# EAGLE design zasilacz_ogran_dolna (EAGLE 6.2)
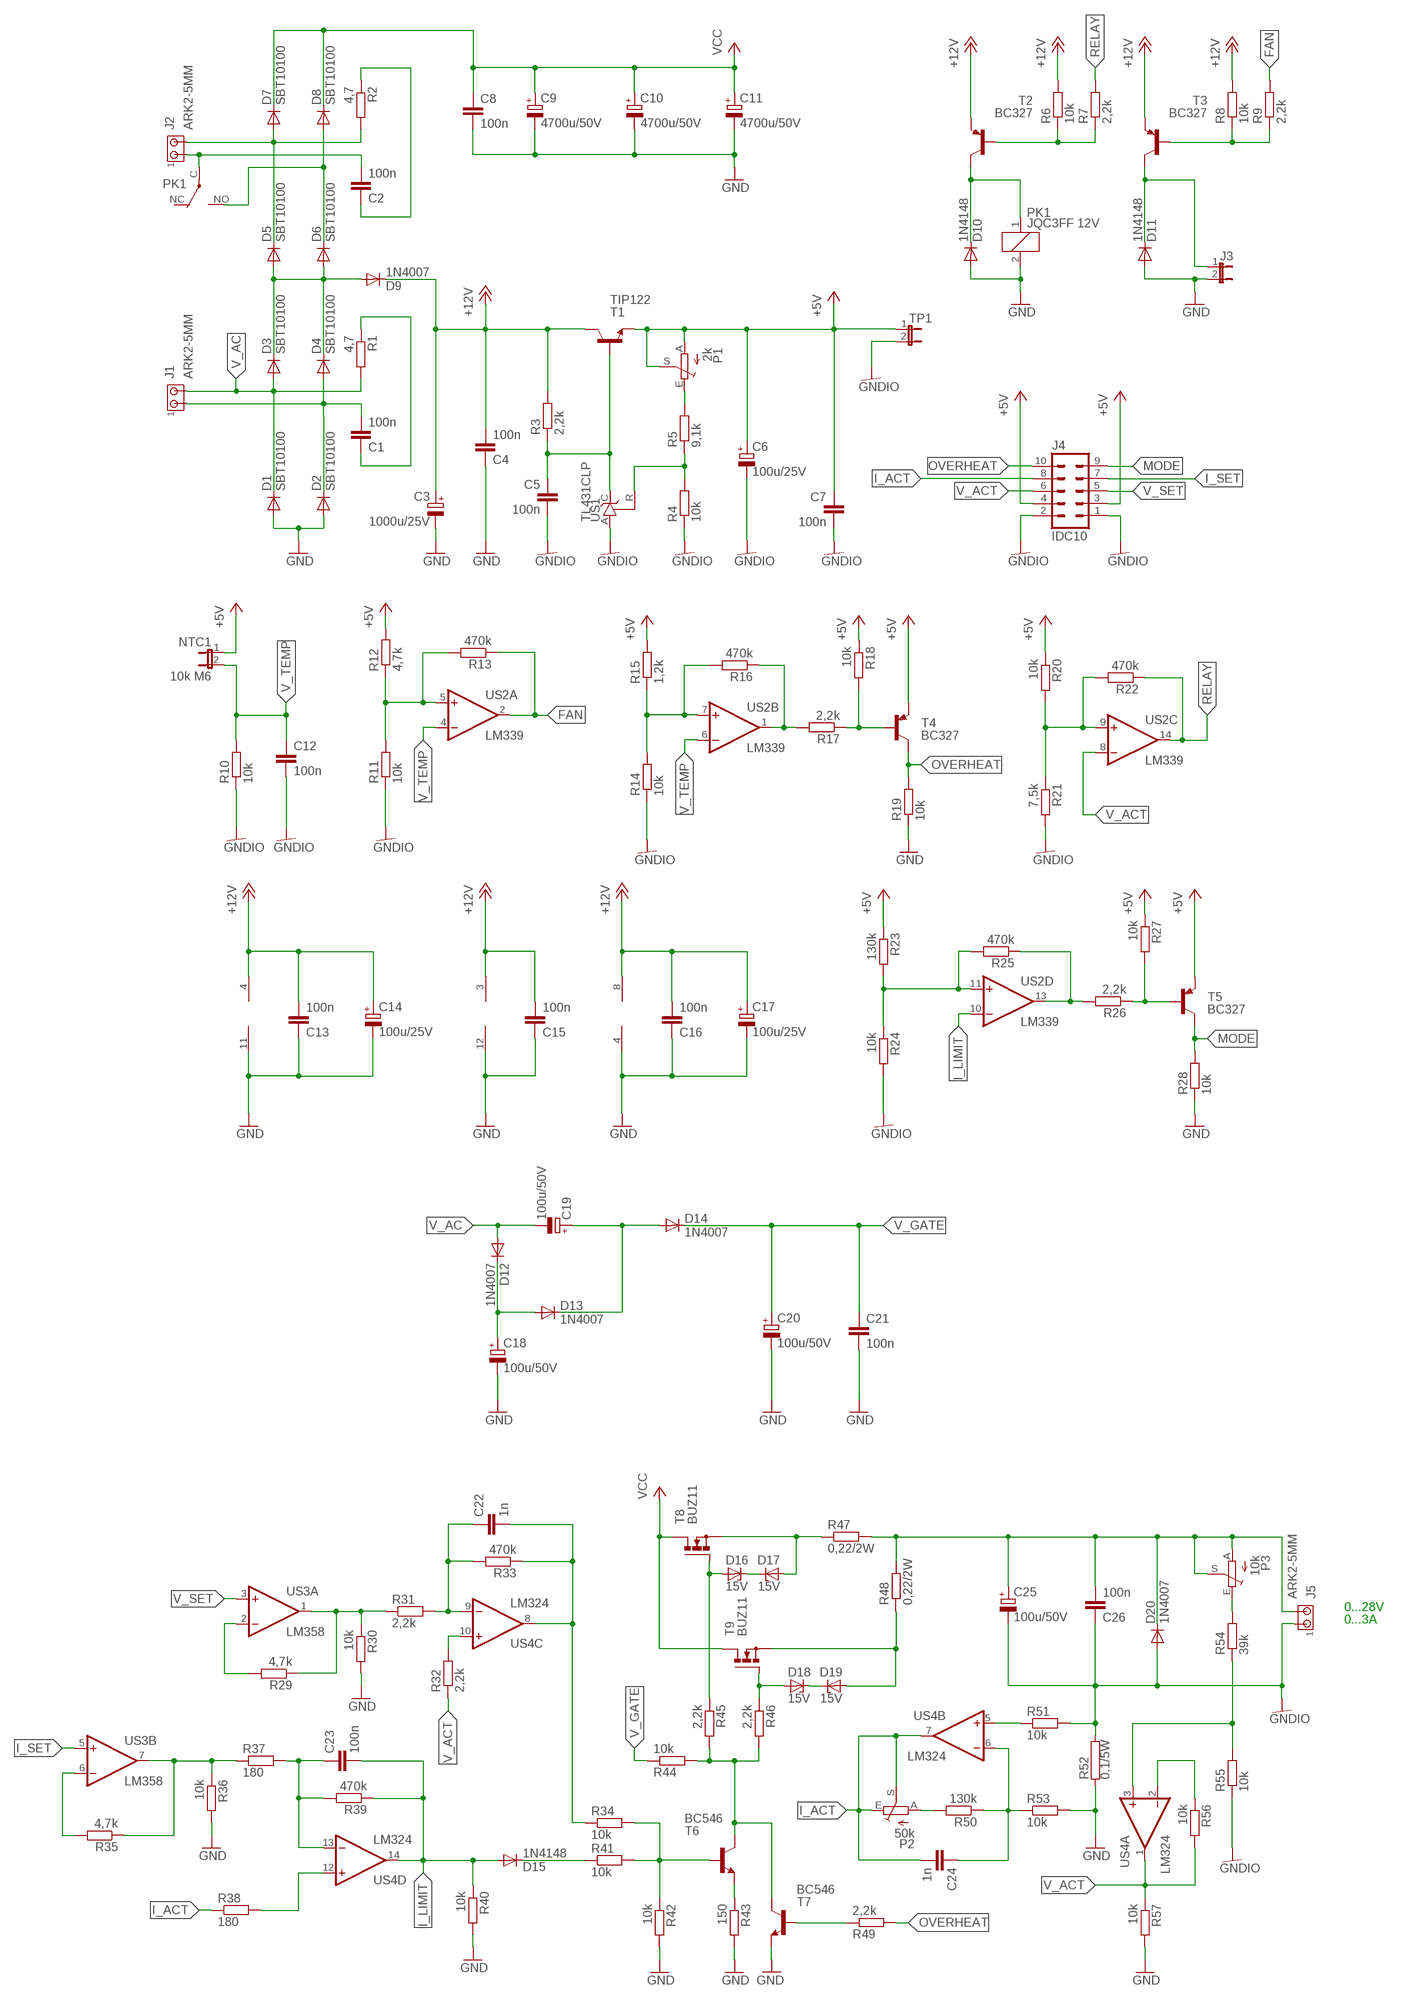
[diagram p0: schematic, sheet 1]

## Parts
C1  100n  C-EU050-025X075  [C050-025X075]
C2  100n  C-EU050-025X075  [C050-025X075]
C3  1000u/25V  CPOL-EUE5-10.5  [E5-10,5]
C4  100n  C-EU050-025X075  [C050-025X075]
C5  100n  C-EU050-025X075  [C050-025X075]
C6  100u/25V  CPOL-EUE2.5-6  [E2,5-6]
C7  100n  C-EU050-025X075  [C050-025X075]
C8  100n  C-EU050-025X075  [C050-025X075]
C9  4700u/50V  CPOL-EUE10-20  [EB20D]
C10  4700u/50V  CPOL-EUE10-20  [EB20D]
C11  4700u/50V  CPOL-EUE10-20  [EB20D]
C12  100n  C-EU050-025X075  [C050-025X075]
C13  100n  C-EU050-025X075  [C050-025X075]
C14  100u/25V  CPOL-EUE2.5-6  [E2,5-6]
C15  100n  C-EU050-025X075  [C050-025X075]
C16  100n  C-EU050-025X075  [C050-025X075]
C17  100u/25V  CPOL-EUE2.5-6  [E2,5-6]
C18  100u/50V  CPOL-EUE3.5-8  [E3,5-8]
C19  100u/50V  CPOL-EUE3.5-8  [E3,5-8]
C20  100u/50V  CPOL-EUE3.5-8  [E3,5-8]
C21  100n  C-EU050-025X075  [C050-025X075]
C22  1n  C-EU050-025X075  [C050-025X075]
C23  100n  C-EU050-025X075  [C050-025X075]
C24  1n  C-EU050-025X075  [C050-025X075]
C25  100u/50V  CPOL-EUE3.5-8  [E3,5-8]
C26  100n  C-EU050-025X075  [C050-025X075]
D1  SBT10100  DIODE-TO220V  [TO220ACS]
D2  SBT10100  DIODE-TO220V  [TO220ACS]
D3  SBT10100  DIODE-TO220V  [TO220ACS]
D4  SBT10100  DIODE-TO220V  [TO220ACS]
D5  SBT10100  DIODE-TO220V  [TO220ACS]
D6  SBT10100  DIODE-TO220V  [TO220ACS]
D7  SBT10100  DIODE-TO220V  [TO220ACS]
D8  SBT10100  DIODE-TO220V  [TO220ACS]
D9  1N4007  DIODE-DO41-7.6  [DO41-7.6]
D10  1N4148  DIODE-DO34-7  [DO34-7]
D11  1N4148  DIODE-D-5  [D-5]
D12  1N4007  1N4004  [DO41-10]
D13  1N4007  1N4004  [DO41-10]
D14  1N4007  1N4004  [DO41-10]
D15  1N4148  DIODE-DO34-7  [DO34-7]
D16  15V  ZENER-DIODEDO34-7  [DO34Z7]
D17  15V  ZENER-DIODEDO34-7  [DO34Z7]
D18  15V  ZENER-DIODEDO34-7  [DO34Z7]
D19  15V  ZENER-DIODEDO34-7  [DO34Z7]
D20  1N4007  DIODE-DO41-7.6  [DO41-7.6]
J1  ARK2-5MM  [2PIN-5MM]
J2  ARK2-5MM  [2PIN-5MM]
J3  JP1E  [JP1]
J4  IDC10  ML10  [ML10]
J5  ARK2-5MM  [2PIN-5MM]
NTC1  10k M6  JP1E  [JP1]
P1  2k  TRIM_EU-B64Y  [B64Y]
P2  50k  TRIM_EU-B64Y  [B64Y]
P3  10k  TRIM_EU-B64Y  [B64Y]
PK1  JQC3FF 12V  PK_POJED-JQC-3FG  [PK_POJED_JQC-3FG]
R1  4,7  R-EU_0207/7  [0207/7]
R2  4,7  R-EU_0207/7  [0207/7]
R3  2,2k  R-EU_0207/7  [0207/7]
R4  10k  R-EU_0207/7  [0207/7]
R5  9,1k  R-EU_0207/7  [0207/7]
R6  10k  R-EU_0207/7  [0207/7]
R7  2,2k  R-EU_0207/7  [0207/7]
R8  10k  R-EU_0207/7  [0207/7]
R9  2,2k  R-EU_0207/7  [0207/7]
R10  10k  R-EU_0207/7  [0207/7]
R11  10k  R-EU_0207/7  [0207/7]
R12  4,7k  R-EU_0207/7  [0207/7]
R13  470k  R-EU_0207/7  [0207/7]
R14  10k  R-EU_0207/7  [0207/7]
R15  1,2k  R-EU_0207/7  [0207/7]
R16  470k  R-EU_0207/7  [0207/7]
R17  2,2k  R-EU_0207/7  [0207/7]
R18  10k  R-EU_0207/7  [0207/7]
R19  10k  R-EU_0207/7  [0207/7]
R20  10k  R-EU_0207/7  [0207/7]
R21  7,5k  R-EU_0207/7  [0207/7]
R22  470k  R-EU_0207/7  [0207/7]
R23  130k  R-EU_0207/7  [0207/7]
R24  10k  R-EU_0207/7  [0207/7]
R25  470k  R-EU_0207/7  [0207/7]
R26  2,2k  R-EU_0207/7  [0207/7]
R27  10k  R-EU_0207/7  [0207/7]
R28  10k  R-EU_0207/7  [0207/7]
R29  4,7k  R-EU_0207/7  [0207/7]
R30  10k  R-EU_0207/7  [0207/7]
R31  2,2k  R-EU_0207/7  [0207/7]
R32  2,2k  R-EU_0207/7  [0207/7]
R33  470k  R-EU_0207/7  [0207/7]
R34  10k  R-EU_0207/7  [0207/7]
R35  4,7k  R-EU_0207/7  [0207/7]
R36  10k  R-EU_0207/7  [0207/7]
R37  180  R-EU_0207/7  [0207/7]
R38  180  R-EU_0207/7  [0207/7]
R39  470k  R-EU_0207/7  [0207/7]
R40  10k  R-EU_0207/7  [0207/7]
R41  10k  R-EU_0207/7  [0207/7]
R42  10k  R-EU_0207/7  [0207/7]
R43  150  R-EU_0207/7  [0207/7]
R44  10k  R-EU_0207/7  [0207/7]
R45  2,2k  R-EU_0207/7  [0207/7]
R46  2,2k  R-EU_0207/7  [0207/7]
R47  0,22/2W  R-EU_0817/7V  [P0817V]
R48  0,22/2W  R-EU_0817/7V  [P0817V]
R49  2,2k  R-EU_0207/7  [0207/7]
R50  130k  R-EU_0207/7  [0207/7]
R51  10k  R-EU_0207/7  [0207/7]
R52  0,1/5W  R-5W  [R_5W]
R53  10k  R-EU_0207/7  [0207/7]
R54  39k  R-EU_0207/7  [0207/7]
R55  10k  R-EU_0207/7  [0207/7]
R56  10k  R-EU_0207/7  [0207/7]
R57  10k  R-EU_0207/7  [0207/7]
T1  TIP122  -NPN-TO220V  [TO220V]
T2  BC327  BC556  [TO92-EBC]
T3  BC327  BC556  [TO92-EBC]
T4  BC327  BC556  [TO92-EBC]
T5  BC327  BC556  [TO92-EBC]
T6  BC546  BC546A  [TO92-EBC]
T7  BC546  BC546A  [TO92-EBC]
T8  BUZ11  BUZ11BV  [TO220BV]
T9  BUZ11  BUZ11BV  [TO220BV]
TP1  JP1E  [JP1]
US1  TL431CLP  [TO92-CLP]
US2  LM339  LM339N  [DIL14]
US3  LM358  LM358N  [DIL08]
US4  LM324  LM324N  [DIL14]

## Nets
+5V: C6.+ C7.1 J4.3 J4.4 NTC1.1 P1.A P1.S R12.2 R15.2 R18.1 R20.1 R23.1 R27.1 T1.3(E) T4.E T5.E TP1.1
+12V: C3.+ C4.2 C13.2 C14.+ C15.2 C16.2 C17.+ D9.C R3.2 R6.2 R8.2 T1.2(C) T2.E T3.E US2.3(P:V+) US3.8(P:V+) US4.4(P:V+)
FAN: R9.2 R13.1 US2.2(A:OUT)
GND: C3.- C4.1 C8.2 C9.- C10.- C11.- C13.1 C14.- C15.1 C16.1 C17.- C18.- C20.- C21.2 D1.A D2.A D10.A D11.A J3.2 PK1.2 R19.1 R28.1 R30.2 R36.2 R40.2 R42.2 R43.2 R52.P$1 R53.2 R57.2 T7.E US2.12(P:GND) US3.4(P:V-) US4.11(P:V-)
GNDIO: C5.2 C6.- C7.2 C12.2 C25.- C26.1 D20.A J4.1 J4.2 J5.P$1 R4.1 R10.1 R11.1 R14.1 R21.2 R24.2 R51.2 R52.P$2 R55.1 TP1.2 US1.A
I_ACT: C24.2 J4.8 P2.E P2.S R38.1 US4.7(B:OUT)
I_LIMIT: C23.2 D15.A R39.1 R40.1 US2.10(D:-IN) US4.14(D:OUT)
I_SET: J4.7 US3.5(B:+IN)
MODE: J4.9 R28.2 T5.C
N$1: D17.A R47.1 T8.S
N$2: R16.1 R17.2 US2.1(B:OUT)
N$3: C1.1 R1.1
N$4: R11.2 R12.1 R13.2 US2.5(A:+IN)
N$5: R17.1 R18.2 T4.B
N$6: R14.2 R15.1 R16.2 US2.7(B:+IN)
N$7: D19.A R48.1 T9.S
N$8: C5.1 R3.1 T1.1(B) US1.C
N$9: C19.+ D13.C D14.A
N$10: C1.2 D2.C D4.A J1.P$1
N$11: C25.+ C26.2 D20.C J5.P$2 P3.A P3.S R47.2 R48.2
N$12: C18.+ D12.C D13.A
N$13: D16.A R45.1 T8.G
N$14: P3.E R54.2
N$15: D15.C R41.1
N$16: C22.1 R31.2 R33.2 US4.9(C:-IN)
N$17: C24.1 R50.1 R53.1 US4.6(B:-IN)
N$18: P2.A R50.2
N$19: R43.1 T6.E
N$20: C22.2 R33.1 R34.1 US4.8(C:OUT)
N$21: R54.1 R55.2 US4.3(A:+IN)
N$22: R32.2 US4.10(C:+IN)
N$23: P1.E R5.2
N$24: C2.1 R2.1
N$25: D10.C PK1.1 T2.C
N$26: D3.C D4.C D5.A D6.A D9.A
N$27: D5.C D7.A J2.P$2 R2.2
N$28: D6.C D8.A PK1.NO
N$29: R6.1 R7.1 T2.B
N$30: D11.C J3.1 T3.C
N$31: C2.2 J2.P$1 PK1.C(COM)
N$32: R8.1 R9.1 T3.B
N$33: R4.2 R5.1 US1.R
N$35: R49.1 T7.B
N$36: C23.1 R37.2 R39.2 US4.13(D:-IN)
N$37: R25.1 R26.2 US2.13(D:OUT)
N$39: R26.1 R27.2 T5.B
N$40: R23.2 R24.1 R25.2 US2.11(D:+IN)
N$41: R20.2 R21.1 R22.2 US2.9(C:+IN)
N$47: D16.C D17.C
N$48: R44.2 R45.2 R46.2 T6.C T7.C
N$49: D18.A R46.1 T9.G
N$50: D18.C D19.C
N$52: R34.2 R41.2 R42.1 T6.B
N$53: R51.1 US4.5(B:+IN)
N$54: R29.2 US3.2(A:-IN)
N$58: R38.2 US4.12(D:+IN)
N$59: R35.2 US3.6(B:-IN)
N$60: R29.1 R30.1 R31.1 US3.1(A:OUT)
N$61: R56.1 US4.2(A:-IN)
N$62: R35.1 R36.1 R37.1 US3.7(B:OUT)
OVERHEAT: J4.10 R19.2 R49.2 T4.C
RELAY: R7.2 R22.1 US2.14(C:OUT)
V_AC: C19.- D1.C D3.A D12.A J1.P$2 R1.2
V_ACT: J4.6 R32.1 R56.2 R57.1 US2.8(C:-IN) US4.1(A:OUT)
V_GATE: C20.+ C21.1 D14.C R44.1
V_SET: J4.5 US3.3(A:+IN)
V_TEMP: C12.1 NTC1.2 R10.2 US2.4(A:-IN) US2.6(B:-IN)
VCC: C8.1 C9.+ C10.+ C11.+ D7.C D8.C T8.D T9.D
Unconnected: PK1.NC

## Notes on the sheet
- 0...28V
- 0...3A

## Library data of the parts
C1 C2 C4 C5 C7 C8 C12 C13 C15 C16 C21-C24 C26 = rcl:C-EU: CAPACITOR, European symbol
C3 C6 C9-C11 C14 C17-C20 C25 = rcl:CPOL-EU: POLARIZED CAPACITOR, European symbol
D1-D11 D15 D20 = diode:DIODE-: DIODE
D12-D14 = diode:1N4004: DIODE
D16-D19 = diode:ZENER-DIODE: Z-Diode
J1 J2 J5 = zlacza_futrzak:ARK2: ARK 2
J3 NTC1 TP1 = jumper:JP1E: JUMPER
J4 = con-ml:ML10: HARTING; OC_FARNELL: unknown; OC_NEWARK: unknown
P1-P3 = pot:TRIM_EU-: POTENTIOMETER
PK1 = inne_futrzak:PK_POJED
R1-R51 R53-R57 = rcl:R-EU_: RESISTOR, European symbol
R52 = inne_futrzak:R
T1 = transistor:*-NPN-: NPN Transistror BF959 corrected 2008.03.06
T2-T5 = transistor-pnp:BC556*: PNP Transistror
T6 T7 = transistor-npn:BC546*: NPN Transistor
T8 T9 = transistor-power:BUZ11: N-CHANNEL MOS FET
US1 = v-reg:TL431CLP: VOLTAGE REGULATOR
US2 = linear:LM339: Low Power Low Offset Voltage Quad Comparators with open collector; LM139/LM239/LM339/LM2901/LM3302
US3 = linear:LM358: OP AMP also LM158; LM258; LM2904 Source: http://cache.national.com/ds/LM/LM158.pdf
US4 = linear:LM324: OP AMP

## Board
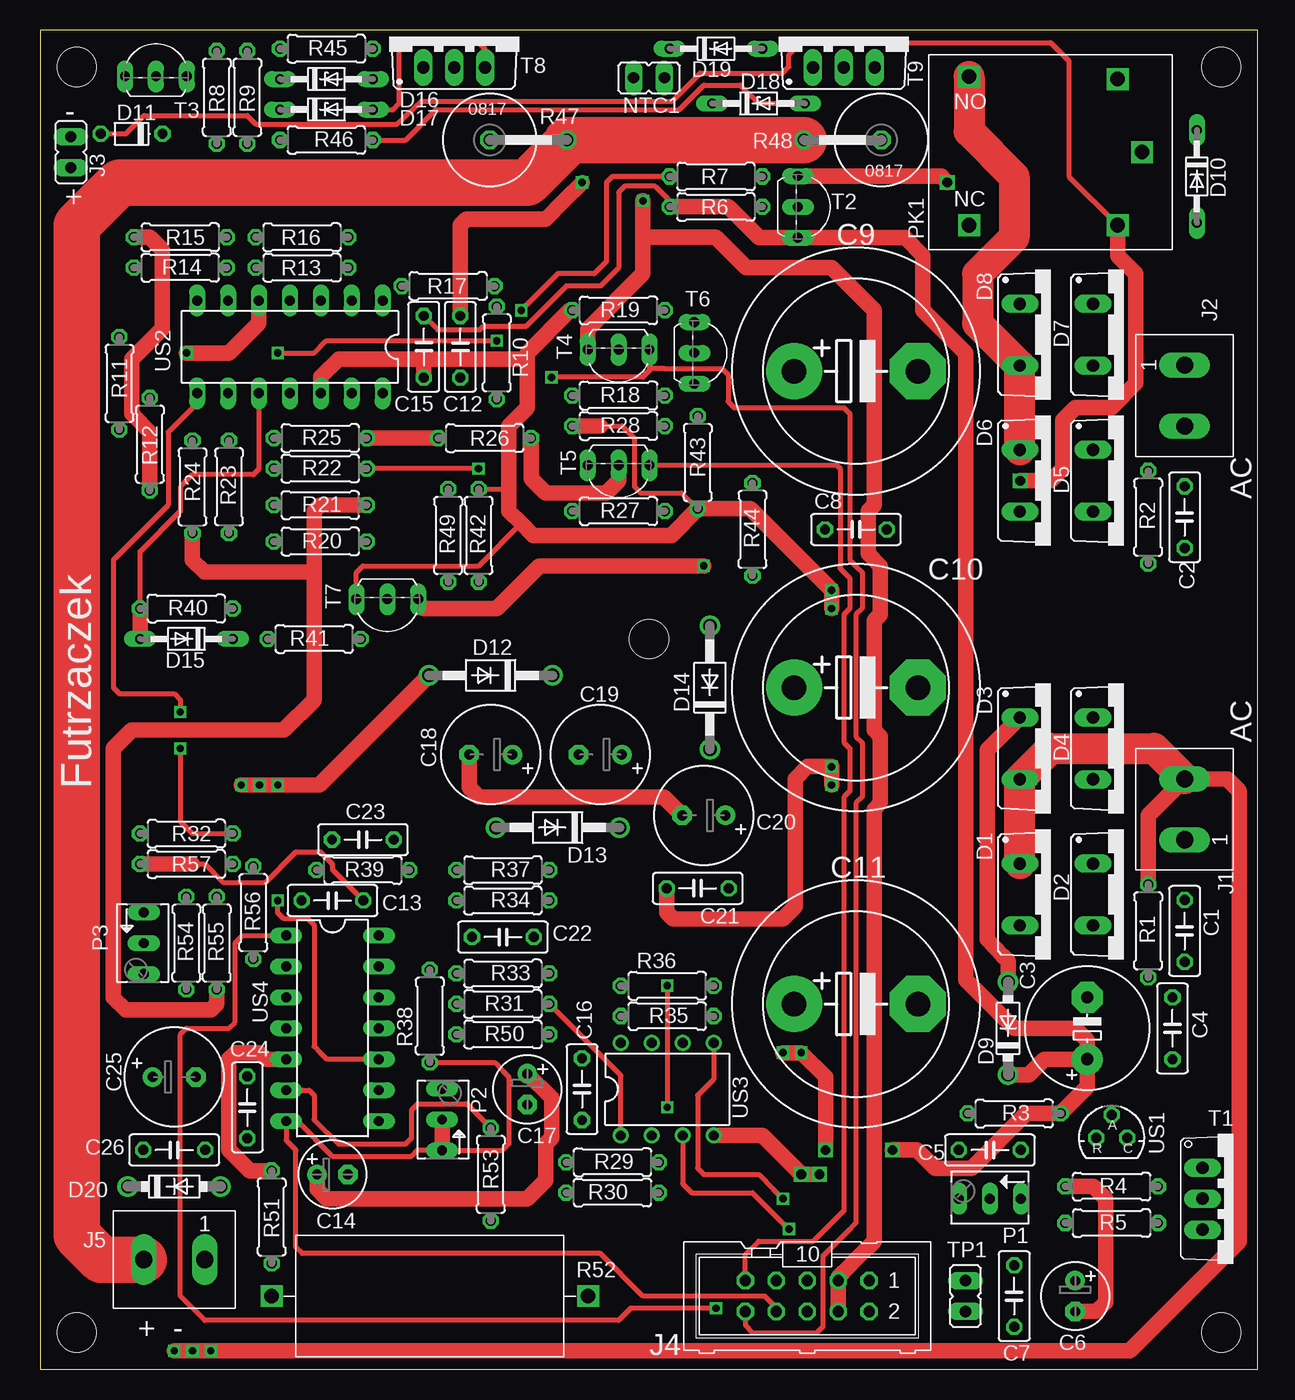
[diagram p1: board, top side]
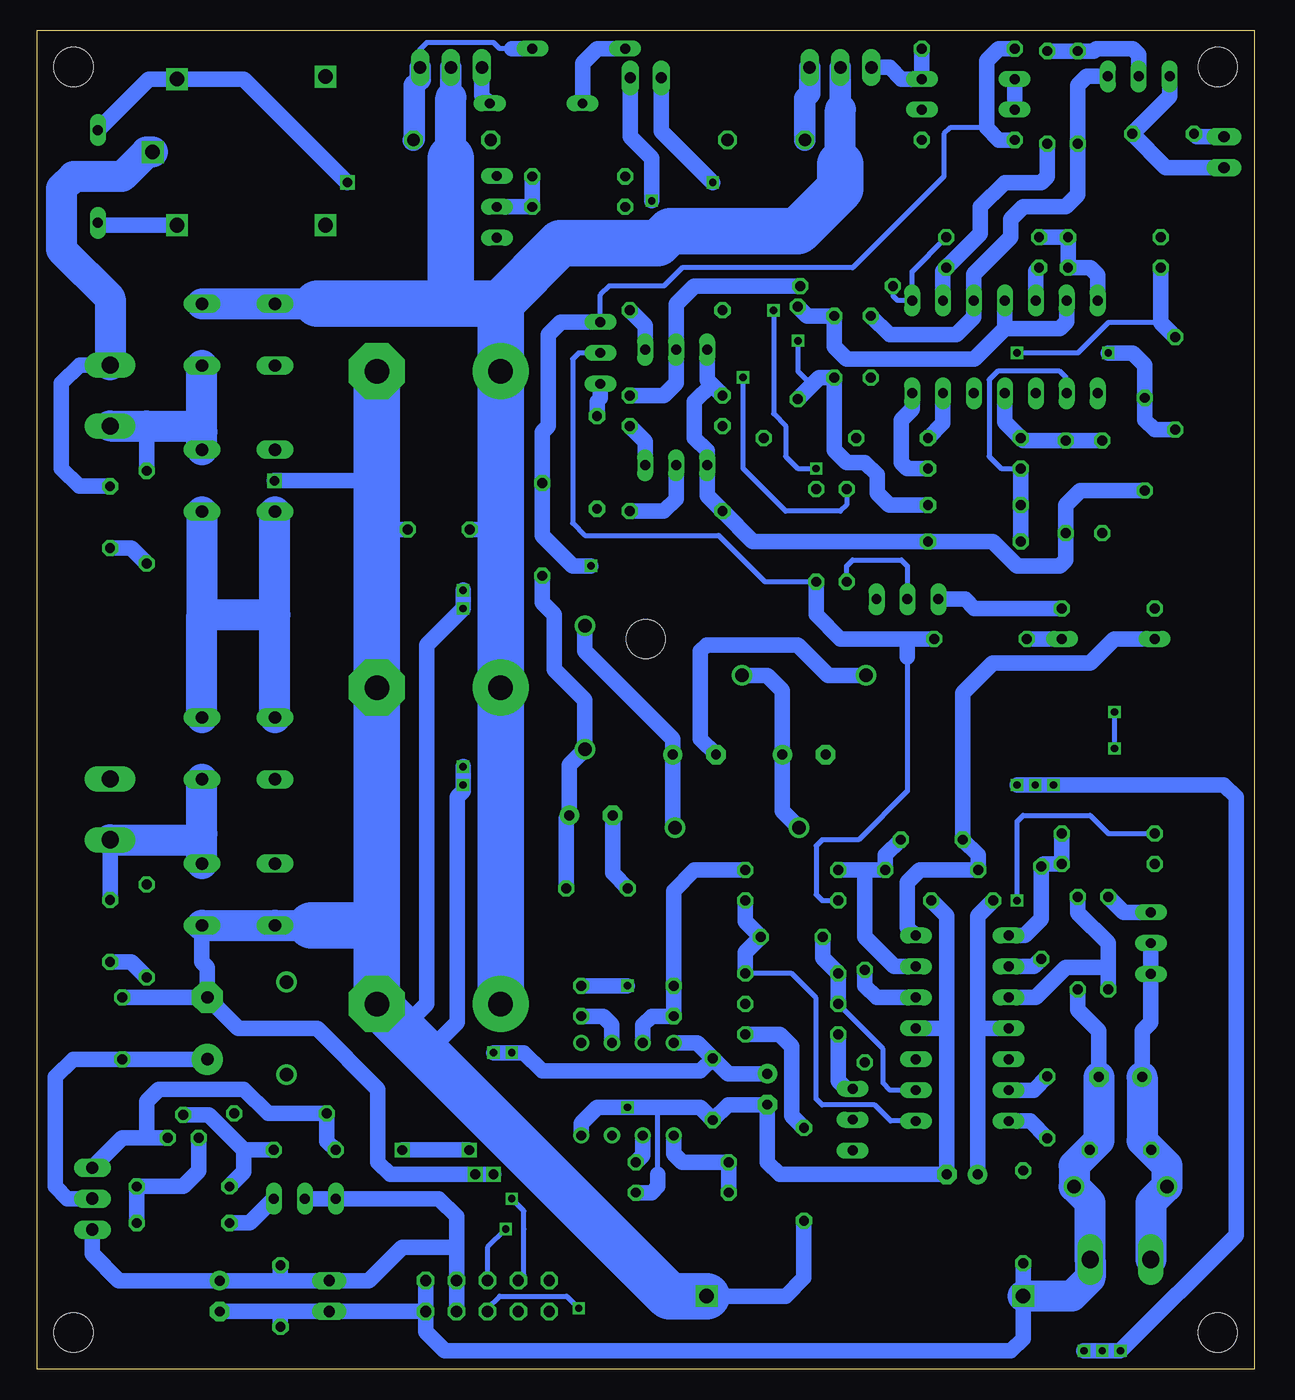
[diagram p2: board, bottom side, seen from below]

Size 100 x 110 mm. Coordinates in mm from the lower left corner, seen from the top.
Outline: 0,0 100,0 100,110 0,110 0,0
Copper layers (1*16): Top 0.035mm / dielectric 1.5mm / Bottom 0.035mm
Design rules: minimum track width 10mil, minimum drill 23mil, track to track 8mil, track to pad 8mil, pad to pad 8mil, via to via 8mil, smd to smd 8mil, copper to edge 20mil, drill to drill 8mil, minimum pad ring 10mil, minimum via ring 8mil, stop-mask expansion 4mil, vias tented up to drill 0mil, thermal gap 10mil
Holes 3.2 mm at 3,3 97,3 3,107 97,107 50,60

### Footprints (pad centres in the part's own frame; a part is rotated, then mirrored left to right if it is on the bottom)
C050-025X075 = drill 0.813 octagon: 1 -2.54,0; 2 2.54,0
E5-10,5 = drill 1.016 pad 2.54: + -2.54,0 | drill 1.016 pad 2.54 octagon: - 2.54,0
E2,5-6 = drill 0.813 pad 1.6: + -1.27,0 | drill 0.813 pad 1.6 octagon: - 1.27,0
EB20D = drill 2.007 pad 4.597: + -5.08,0 | drill 2.007 pad 4.597 octagon: - 5.08,0
E3,5-8 = drill 0.813 pad 1.6: + -1.778,0 | drill 0.813 pad 1.6 octagon: - 1.778,0
TO220ACS = drill 1.016 long: A 2.54,-2.54; C -2.54,-2.54
DO41-7.6 = drill 1.1 pad 1.7: A 3.81,0; C -3.81,0
DO34-7 = drill 0.813 long: A 3.81,0; C -3.81,0
D-5 = drill 0.813 octagon: A 2.54,0; C -2.54,0
DO41-10 = drill 1.118: A 5.08,0; C -5.08,0
DO34Z7 = drill 0.813 long: A 3.81,0; C -3.81,0
2PIN-5MM = drill 1.4 long: P$1 -2.5,0; P$2 2.5,0
JP1 = drill 0.914 long: 1 0,-1.27; 2 0,1.27
ML10 = drill 0.914 octagon: 1 -5.08,-1.27; 2 -5.08,1.27; 3 -2.54,-1.27; 4 -2.54,1.27; 5 0,-1.27; 6 0,1.27; 7 2.54,-1.27; 8 2.54,1.27; 9 5.08,-1.27; 10 5.08,1.27
B64Y = drill 0.813 long: A 2.54,0; E -2.54,0; S 0,0
PK_POJED_JQC-3FG = drill 1.2 square: 1 5.5,6; 2 5.5,-6; C 7.5,0; NC -6.7,-6; NO -6.7,6.2
0207/7 = drill 0.813 octagon: 1 -3.81,0; 2 3.81,0
P0817V = drill 1.016 octagon: 1 -5.08,0; 2 1.27,0
R_5W = drill 1.2 square: P$1 -13,0; P$2 13,0
TO220V = drill 1.016 long: 1 -2.54,-2.54; 2 0,-2.54; 3 2.54,-2.54
TO92-EBC = drill 0.813 long: B 0,-1.27; C -2.54,-1.27; E 2.54,-1.27
TO220BV = drill 1.016 long: D 0,-2.54; G -2.54,-2.54; S 2.54,-2.54
TO92-CLP = drill 0.813 octagon: A 0,1.905; C 1.27,0; R -1.27,0
DIL14 = drill 0.813 long: 1 -7.62,-3.81; 2 -5.08,-3.81; 3 -2.54,-3.81; 4 0,-3.81; 5 2.54,-3.81; 6 5.08,-3.81; 7 7.62,-3.81; 8 7.62,3.81; 9 5.08,3.81; 10 2.54,3.81; 11 0,3.81; 12 -2.54,3.81; 13 -5.08,3.81; 14 -7.62,3.81
DIL08 = drill 0.813 pad 1.27: 1 -3.81,-3.81; 2 -1.27,-3.81; 3 1.27,-3.81; 4 3.81,-3.81; 5 3.81,3.81; 6 1.27,3.81; 7 -1.27,3.81; 8 -3.81,3.81

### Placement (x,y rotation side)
C1  94,36 90 top
C2  94,70 90 top
C3  86,28 90 top
C4  93,28 270 top
C5  78,18 0 top
C6  85,6 270 top
C7  80,6 270 top
C8  67,69 0 top
C9  67,82 0 top
C10  67,56 0 top
C11  67,30 0 top
C12  34.5,84 270 top
C13  24,38.5 180 top
C14  24,16 0 top
C15  31.5,84 90 top
C16  44.5,23 90 top
C17  40,23 270 top
C18  37,50.5 180 top
C19  46,50.5 180 top
C20  54.5,45.5 180 top
C21  54,39.5 180 top
C22  38,35.5 0 top
C23  26.5,43.5 180 top
C24  17,21.5 270 top
C25  11,24 0 top
C26  11,18 180 top
D1  83,39 270 top
D2  89,39 270 top
D3  83,51 270 top
D4  89,51 270 top
D5  89,73 270 top
D6  83,73 270 top
D7  89,85 270 top
D8  83,85 270 top
D9  79.5,28 90 top
D10  95,98 270 top
D11  7.5,101.5 180 top
D12  37,57 180 top
D13  42.5,44.5 180 top
D14  55,56 90 top
D15  12,60 180 top
D16  23.5,106 0 top
D17  23.5,103.5 0 top
D18  59,104 0 top
D19  55.5,108.5 0 top
D20  11,15 0 top
J1  94,46 90 top
J2  94,80 270 top
J3  2.5,100 0 top
J4  63,6 180 top
J5  11,9 180 top
NTC1  50,106.1 90 top
P1  78,14 180 top
P2  33,20.5 90 top
P3  8.5,35 270 top
PK1  83,100 0 top
R1  91,36 90 top
R2  91,70 90 top
R3  80,21 0 top
R4  88,15 0 top
R5  88,12 180 top
R6  55.5,95.5 180 top
R7  55.5,98 180 top
R8  14.5,104.5 270 top
R9  17,104.5 270 top
R10  37.5,83.5 90 top
R11  6.5,81 270 top
R12  9,76 270 top
R13  21.5,90.5 180 top
R14  11.5,90.5 0 top
R15  11.5,93 180 top
R16  21.5,93 180 top
R17  33.5,89 180 top
R18  47.5,80 0 top
R19  47.5,87 0 top
R20  23,68 180 top
R21  23,71 0 top
R22  23,74 180 top
R23  15.5,72.5 90 top
R24  12.5,72.5 270 top
R25  23,76.5 180 top
R26  36.5,76.5 180 top
R27  47.5,70.5 0 top
R28  47.5,77.5 0 top
R29  47,17 0 top
R30  47,14.5 0 top
R31  38,30 180 top
R32  12,44 180 top
R33  38,32.5 180 top
R34  38,38.5 180 top
R35  51.5,29 0 top
R36  51.5,31.5 0 top
R37  38,41 180 top
R38  32,29 90 top
R39  26.5,41 0 top
R40  12,62.5 0 top
R41  22.5,60 0 top
R42  36,68.5 90 top
R43  54,74.5 270 top
R44  58.5,69 90 top
R45  23.5,108.5 180 top
R46  23.5,101 180 top
R47  42,101 0 top
R48  64,101 180 top
R49  33.5,68.5 90 top
R50  38,27.5 180 top
R51  19,12.5 270 top
R52  32,6 180 top
R53  37,16 270 top
R54  12,35 90 top
R55  14.5,35 90 top
R56  17.5,37.5 90 top
R57  12,41.5 180 top
T1  98,14 270 top
T2  63.5,95.5 270 top
T3  9.5,107.5 0 top
T4  47.5,82.5 180 top
T5  47.5,73 180 top
T6  55,83.5 270 top
T7  28.5,62 180 top
T8  34,109.5 0 top
T9  66,109.5 0 top
TP1  76,6 180 top
US1  88,19 0 top
US2  20.5,84 180 top
US3  51.5,23 0 top
US4  24,28 270 top

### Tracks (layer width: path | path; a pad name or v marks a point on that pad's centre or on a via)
+5V  (via drill 0.6)
  Top 1.27: J4.4 65.54,7.54 66,8 67.25,9.25 | v49.5,96 49.5,94 49.5,93 | 65.25,90.25 65,90.5 58,90.5 55.5,93 50.5,93 49.5,93 | 65.25,90.25 66,89.5 | R15.2 9,93 10,92 10,85.5 8,83.5 7.5,83 7.5,78.5 9,77 R12.2 | 67.25,9.25 68,10 68.5,10.5 | 65.25,90.25 68.5,87 68.5,71 68,70.5 68,67 69,66 69,62 68.5,61.5 68.5,52.5 69,52 69,46.5 68.5,46 68.5,10.5 | 68.5,10.5 67.25,9.25 | T4.E 44.96,85.46 49.5,90 49.5,93
  Bottom 1.27: T1.3 95.46,9.46 93.27,7.27 C6.+ 80,7.27 | 80,7.27 TP1.1 72.73,7.27 70,10 65.54,10 | C7.1 80,7.27 | J4.4 J4.3 65.54,10 | 65.54,10 65.54,12.54 67,14 P1.A P1.S | R12.2 14.31,72.19 15.5,71 R23.1 15.5,66.5 16,66 19.5,66 21.5,68 R20.1 41.19,68 R27.1 44.96,71.77 T5.E 44.96,75.46 46,76.5 46,79.5 44.59,80.91 | NTC1.1 51.27,101.27 49.5,99.5 v49.5,96 | T4.E 44.96,81.27 44.59,80.91 | 44.59,80.91 R18.1
+12V  (via drill 0.6, 0.8)
  Top 0.406: 51.69,95.81 R6.2 51.69,96.01 50.5,97.2 48,97.2 47.5,96.7 47.5,90.5 46,89 43.2,89 39.9,85.7 36.4,85.7 36.1,85.4 32.64,85.4 C15.2
  Top 1.27: C3.+ 86,23.19 R3.2 81,21 76.5,16.5 73.5,16.5 72,18 v70,18 | R6.2 56.5,95.5 59.04,92.96 T2.E 71.04,92.96 72.5,91.5 72.5,87 76,83.5 76,32 79,29 79.5,28.5 80,28 85,28 86,27 C3.+ | v64.5,18 64.5,24 v62.5,26 v61,26 | C14.+ 22.73,14.77 23.5,14 40,14 41.5,15.5 41.5,18.5 42,19 42,22.27 C17.+ | D9.C 81.19,24.19 82,25 82.46,25.46 C3.+
  Bottom 1.27: T1.2 97.5,14 98.5,15 98.5,24 97.04,25.46 C4.2 C3.+ 85.73,25.19 | C15.2 29.96,85 24.5,85 23.04,86.46 US2.3 23.04,89.96 20,93 20,94.5 19,95.5 15.5,95.5 14.5,96.5 R8.2 14.5,105.5 13.77,106.23 T3.E | 22.73,28 22.73,37.23 C13.2 | US4.4 22.73,28 | v64.5,18 v70,18 | v62.5,26 60,26 58.5,24.5 45.5,24.5 44.5,25.5 C16.2 | C17.+ 43.23,24.27 C16.2 | US3.8 45.77,26.81 C16.2 | 22.73,28 C14.+
FAN
  Bottom 1.27: US2.2 25.58,90.23 R13.1 22.5,93.31 22.5,95.5 20.5,97.5 17.5,97.5 17,98 R9.2
GND  (via drill 0.6, 0.8)
  Top 0.406: 46,77.5 47.8,77.5 48.8,76.5 48.8,72.5 49.3,72 52.69,72 R43.2 | D11.A 7,101.5 8.5,103 17,103 17.7,102.3 29.3,102.3 31.3,104.2 51.9,104.2 54.2,106.5 61,106.5 61.5,107 61.5,108 62.5,109 83,109 84.5,107.5 84.5,98 PK1.2 | v51.5,31.5 v51.5,21.5 | 12.5,41.5 13.5,41.5 15,40 18.5,40 21,42.5 23,42.5 24,41.5 24,41.04 C13.1 | R42.2 38.31,72.31 38.5,72.5 | T7.E 25.96,65.46 26.5,66 36,66 39.5,69.5
  Top 1.27: PK1.2 88.5,91.5 90,90 90,81 88,79 85,79 84,78 84,74 83,73 v80.5,73 | US2.12 23.04,81.54 24.5,83 31.5,83 | R28.1 46,77.5 | R19.1 43.5,87 40,83.5 40,83 | 31.5,83 40,83 | C15.1 31.5,83 | v65,62.5 v65,64 58.31,70.69 R43.2 51.81,68.5 40.5,68.5 39.5,69.5 38.5,70.5 38.5,72.5 38.5,77.5 40,79 40,83 | v65,48 v65,49.5 63,49.5 62,48.5 62,38 61,37 52,37 51.46,37.54 C21.2 | US3.4 59.31,19.19 v62.5,16 v64,16 | R57.2 12.5,41.5 | C18.- 35.22,47.78 36,47 51.22,47 C20.-
  Bottom 0.406: 49,16 49,21.5
  Bottom 1.27: C4.1 C3.- | D2.A 86.46,33.46 86,33 C3.- | v80.5,73 72.08,73 | v62.5,16 71,16 72,17 72,23 77,28 83.46,28 C3.- | C8.2 72.08,69 | PK1.2 94.81,94 D10.A | J3.2 4.73,101.27 D11.A | v65,64 v65,62.5 68,59.5 68,30 70.04,27.96 | v65,49.5 65,47.5 65.5,47 65.5,28.5 68.04,25.96 | C20.- 52.72,40.76 C21.2 | US3.4 55.31,20.19 54,21.5 v51.5,21.5 49,21.5 45.5,21.5 44.5,20.5 C16.1 43.23,21.73 C17.- 40,17 39,16 C14.- 25.27,28 | R30.2 49.5,14.5 49,15 49,16 | R36.2 v51.5,31.5 | 25.27,28 25.27,37.23 C13.1 | US4.11 25.27,28 | R53.2 37,7.5 38.5,6 R52.P$1 | R40.2 23,62.5 23.77,63.27 T7.E
  Bottom 2.54: D2.A D1.A 77.46,36.46
  Bottom 3.81: 72.08,36 C11.- 70.04,27.96 68.04,25.96 48.08,6 R52.P$1 | 72.08,36 C10.- 72.08,69 72.08,73 C9.- | 77.46,36.46 72.54,36.46 72.08,36
GNDIO  (via drill 0.6)
  Top 0.406: v19.5,83.5 22.5,83.5 23.5,84.5 v37.5,84.5
  Top 1.27: C6.- 86.73,4.73 87.5,5.5 87.5,14 86.5,15 R4.1 | R21.2 23,71 22.5,70.5 22.5,65.5 | 22.5,65.5 22.5,55 20,52.5 7.5,52.5 6,51 6,30.5 7,29.5 14,29.5 14.5,30 R55.1 | R24.2 12.5,66.5 13.5,65.5 22.5,65.5
  Bottom 0.406: v37.5,84.5 37.5,82 36.34,80.84 | 7.69,86 12,86 14.5,83.5 v19.5,83.5
  Bottom 1.27: 83,18 85.91,20.91 US1.A | 83,18 83,16.19 R4.1 | J4.1 J4.2 | J4.2 TP1.2 80,4.73 | 80,4.73 C6.- | C7.2 80,4.73 | C5.2 83,18 | R10.1 36.34,80.84 35.73,81.46 C12.2 34.5,75.5 33.5,74.5 32,74.5 31,73.5 31,72 30,71 R21.2 | R14.1 7.69,86 R11.1 | J4.2 68.08,3.08 66.5,1.5 20,1.5 19,2.5 R52.P$2 R51.2 | C25.- 12.78,27.78 14.5,29.5 R55.1
  Bottom 2.54: C25.- 12.78,18.76 C26.1 14.81,16.73 D20.A 13.5,13.69 J5.P$1 13.5,7.5 15,6 R52.P$2
I_ACT
  Top 0.406: J4.8 60.46,5.04 59.5,6 49.5,6 46,9.5 21.5,9.5 21,10 21,18 20.5,18.5 20.19,18.81 US4.7 21.12,20.38 24,17.5 30.5,17.5 31,18 32.96,18 P2.E 37.96,17.96 38,18 38.5,18.5 38.5,24 38,24.5 37.31,25.19 R38.1
  Top 1.27: P2.E P2.S
  Bottom 1.27: US4.7 18.42,20.38 C24.2
I_LIMIT
  Top 0.406: US2.10 17.96,73.96 17.5,73.5 12.5,73.5 11.5,72.5 11.5,70.5 8.19,67.19 R40.1
  Top 1.27: R40.1 D15.A
  Bottom 1.27: US4.14 28.5,36.31 28.5,40 27.5,41 R39.1 22.69,42.23 C23.2 23.96,55.54 21.5,58 13.5,58 11.5,60 D15.A
I_SET  (via drill 0.6)
  Top 0.406: US3.5 55.31,23.81 54,22.5 54,16.5 54.5,16 59,16 60.25,14.75 | 60.25,14.75 v61,14 60.25,14.75
  Bottom 0.406: J4.7 60,7.73 60,11.5 60,13 v61,14
MODE
  Top 0.406: T5.C 65.43,74.27 65.7,74 65.7,65.8 66,65.5 66.5,65 66.5,62.5 66,62 66,51.5 66.5,51 66.5,47.5 66,47 66,13 63.5,10.5 59,10.5 57.92,9.42 J4.9
  Bottom 1.27: T5.C 50.04,76.23 R28.2
N$1
  Top 0.406: D17.A 29,103.5 29.5,104 29.5,108.5 30,109 36,109 36.54,108.46 T8.S
  Bottom 1.778: R47.1 36.92,104.42 36.54,104.8 T8.S
N$2
  Bottom 0.406: R16.1 28.12,90.19 US2.1 29.31,87.81 29.5,88 29.69,88.19 R17.2
N$3
  Bottom 1.27: C1.1 92.27,33.46 R1.1
N$4  (via drill 0.6)
  Top 1.27: v12,83.5 15.5,83.5 16.5,84.5 17.96,85.96 US2.5
  Bottom 1.27: US2.5 17.96,90.23 R13.2 | v12,83.5 10,83.5 9,82.5 R12.1 9,78 8.19,77.19 R11.2
N$5
  Bottom 1.27: R18.2 48.5,80 47.5,81 T4.B 47.5,87.5 46,89 R17.1
N$6
  Bottom 1.27: US2.7 12.88,89.88 13.5,90.5 R14.2 R15.1 R16.2
N$7
  Bottom 0.406: 61,108.5 62,108.5 62.5,109 68,109 68.54,108.46 T9.S
  Bottom 1.27: D19.A 61,108.5
  Bottom 1.778: R48.1 69,101.08 69,105.5 68.54,105.96 T9.S
N$8
  Bottom 1.27: US1.C 91,19 | 91,19 93,19 T1.1 | C5.1 76.19,18.73 R3.1 81,21 83,23 90,23 91,22 91,19
N$9
  Bottom 1.27: D14.A 55,59 47.78,51.78 C19.+ 47.78,44.7 D13.C
N$10
  Bottom 1.27: C1.2 J1.P$1
  Bottom 2.54: D2.C 86.46,44 | 86.46,44 D4.A | J1.P$1 86.96,43.5 86.46,44
N$11
  Top 3.81: J5.P$2 5,9 3,11 3,88.5 3,89 3,94 6.5,97.5 40,97.5 43.27,100.77 R47.2 R48.2
  Bottom 1.27: P3.S P3.A 8.5,28.5 9.22,27.78 C25.+
  Bottom 2.54: J5.P$2 8.5,13.69 D20.C 7.19,16.73 C26.2 9.22,18.76 C25.+
N$12
  Bottom 1.27: D13.A 38.78,45.86 C18.+ 38.78,55.78 40,57 D12.C
N$13
  Bottom 1.27: T8.G 29.96,106.96 29,106 D16.A R45.1
N$14
  Bottom 1.27: P3.E 10.73,37.54 R54.2
N$15
  Bottom 1.27: D15.C R41.1
N$16
  Bottom 0.406: US4.9 29.92,22.92 30.5,23.5 30.5,26.31 R31.2
  Bottom 1.27: C22.1 35.46,33.77 R33.2 R31.2
N$17
  Top 0.406: US4.6 21.58,22.92 22.08,22.92 22.5,22.5 22.5,20.5 24.5,18.5 30,18.5 30.5,19 30.5,21.3 31,21.8 35.01,21.8 R53.1
  Bottom 1.27: US4.6 18.12,22.92 C24.1 | R53.1 38,20.81 38,25 38,26.5 39,27.5 R50.1
N$18
  Bottom 1.27: P2.A 33.54,23.04 34,23.5 34.19,23.69 R50.2
N$19
  Bottom 1.27: T6.E 53.73,79.77 54,79.5 R43.1
N$20
  Bottom 0.406: US4.8 29.88,20.38 31.2,21.7 35.5,21.7 36,22.2 36,30.5 38,32.5 R33.1
  Bottom 1.27: R34.1 41.81,36.77 C22.2 41.81,34.23 R33.1
N$21
  Bottom 1.27: R55.2 14.5,37.5 12,35 12,33 | 12,33 R54.1 | US4.3 17.96,30.54 15.5,33 12,33
N$22  (via drill 0.6)
  Top 0.406: US4.10 23.54,25.46 23,26 22.5,26.5 22.5,36.5 22,37 20,37 19.5,37.5 v19.5,38.5
  Bottom 0.406: v19.5,38.5 19.5,45 19,45.5 13.5,45.5 12,44 R32.2
N$23
  Bottom 1.27: R5.2 82.54,12 P1.E
N$24
  Bottom 1.27: C2.1 92.27,67.46 R2.1
N$25  (via drill 0.8)
  Top 1.27: T2.C 74.04,98.04 v74.5,97.5
  Bottom 1.27: D10.C 90.81,106 PK1.1 83,106 v74.5,97.5
N$26
  Top 1.27: D3.C 77.8,50.88 77.8,35.3 79,34 79.5,33.5 D9.A
  Bottom 2.54: D3.C 80.46,62 | 80.46,62 D6.A | D4.C 86.46,62 | D5.A 86.46,62 | 86.46,62 80.46,62
N$27
  Bottom 1.27: R2.2 91,77.5
  Bottom 2.54: D5.C 86.46,77 | 86.46,77 D7.A | J2.P$2 91,77.5 86.96,77.5 86.46,77
N$28
  Top 2.54: PK1.NO 76.3,101.7 80,98 80,93 77,90 77,85.92 D8.A D6.C
N$29
  Bottom 1.27: T2.B R6.1 R7.1
N$30
  Bottom 1.27: J3.1 7.27,98.73 D11.C 6.96,104.58 T3.C
N$31
  Bottom 1.27: C2.2 96.54,72.54 98,74 98,81 96.5,82.5 J2.P$1
  Bottom 2.54: PK1.C 91,100 93,98 97,98 98,97 98,92 94,88 J2.P$1
N$32
  Bottom 1.27: R9.1 R8.1 13.19,108.31 13,108.5 10,108.5 9.5,108 T3.B
N$33
  Bottom 1.27: R5.1 R4.2 88,15 86.73,16.27 US1.R
N$35
  Bottom 0.406: R49.1 33.5,66 33,66.5 29,66.5 28.5,66 T7.B
N$36
  Bottom 1.27: US4.13 29.58,33.08 32,35.5 32,40.5 32,41 | R37.2 32.5,41 32,41 | 32,41 R39.2 30.31,42.23 C23.1
N$37
  Top 1.27: R25.1 R26.2
  Bottom 1.27: US2.13 25.58,77.73 R25.1
N$39
  Top 1.27: R26.1 40.31,73.19 41.5,72 46.5,72 47.5,73 T5.B
  Bottom 1.27: T5.B 47.5,71.5 48.5,70.5 R27.2
N$40
  Bottom 1.27: US2.11 20.5,77.81 R25.2 19,76.31 R23.2 R24.1
N$41
  Bottom 0.406: US2.9 15.42,81.42 16,82 21.1,82 21.8,81.3 21.8,75 20.8,74 R22.2
  Bottom 1.27: R20.2 R21.1 R22.2
N$47
  Bottom 1.27: D16.C D17.C
N$48  (via drill 0.6)
  Top 1.27: T7.C 31.04,62.96 31.5,62.5 37.5,62.5 41,66 v54.5,66
  Bottom 0.406: 22,102 25,102 25.5,101.5 25.5,98 33,90.5 47,90.5 48.5,89 53,89 53.73,88.27 T6.C
  Bottom 1.27: R46.2 21,101 22,102 22,107.5 21,108.5 R45.2 | T6.C 56.96,86.04 58,85 58,77.5 58.5,77 R44.2 58.5,68.5 56,66 v54.5,66
N$49
  Top 0.406: R46.1 30,101 32.5,103.5 52.5,103.5 54.5,105.5 57.5,105.5 59,104 D18.A
  Bottom 1.27: T9.G 63.46,104.65 D18.A
N$50
  Bottom 1.27: D18.C 55.19,107.31 54,108.5 D19.C
N$52
  Bottom 0.406: T6.B 55.5,83.5 56,83 56,69.5 55,68.5 44,68.5 40.19,64.69 R42.1 | R34.2 35.5,38.5 36,39 36,43 35.5,43.5 32.5,43.5 28.5,47.5 28.5,58.5
  Bottom 1.27: R41.2 28.5,60 | 28.5,58.5 28.5,60 | 28.5,60 34,60 36,62 R42.1
N$53
  Top 1.27: R51.1 17.19,16.31 15.5,18 15.5,25.5 16,26 18,26 18.54,25.46 US4.5
N$54
  Bottom 1.27: US3.2 50.23,17.58 R29.2
N$58
  Bottom 1.27: US4.12 31.04,30.54 32,31.5 R38.2
N$59
  Bottom 1.27: US3.6 52.77,28.27 53.5,29 R35.2
N$60
  Top 0.406: US3.1 47.69,24.12 R31.1
  Bottom 1.27: US3.1 47.69,17.69 47,17 R29.1 R30.1
N$61
  Bottom 1.27: US4.2 18.11,33.08 R56.1
N$62
  Bottom 1.27: US3.7 50.23,28.27 49.5,29 R35.1 R36.1 47.69,39.31 46,41 R37.1
OVERHEAT  (via drill 0.6)
  Top 0.406: T4.C 50.04,83.46 50.04,82.04 | 66.5,11.5 66.25,11.25 | 66.25,11.25 65.5,10.5 64.3,9.3 64.3,3.5 63.8,3 58.5,3 57.92,3.58 J4.10 | 66.25,11.25 67,12 67,46.5 67.5,47 67.5,51.5 67,52 67,62 67.5,62.5 67.5,65.5 67,66 66.5,66.5 66.5,71 66.5,71.5 66.5,78.5 66,79 57,79 56.5,79.5 56.5,81.7 56,82.2 51.3,82.2 50.2,82.2 50.04,82.04 | 50.04,82.04 49.5,81.5 v42,81.5
  Bottom 0.406: R49.2 33.5,71 34,70.5 38.5,70.5 42,74 v42,81.5
  Bottom 1.27: T4.C 50.04,85.73 R19.2
RELAY  (via drill 0.6)
  Top 0.406: R7.2 47,98 46.5,97.5 46.5,94 46.5,91 45.5,90 42.5,90 v39.5,87 | v36,74 R22.1
  Bottom 0.406: v39.5,87 39.5,78.5 38.5,77.5 38.5,75 37.5,74 v36,74
  Bottom 1.27: US2.14 28.12,78.88 29,78 29,74.5 28.5,74 R22.1
V_AC  (via drill 0.6)
  Top 1.27: R1.2 91,45.5 J1.P$2 97.5,48.5 98.5,47.5 98.5,10.5 89.5,1.5 v11,1.5 | D12.A 22.92,48 v19.5,48 v18,48 v16.5,48
  Top 2.54: D1.C D3.A 83,51 91.5,51 J1.P$2
  Bottom 1.27: v14,1.5 v12.5,1.5 v11,1.5 1.5,11 1.5,47 2.5,48 v19.5,48 | D12.A 35,57 37.5,59.5 45,59.5 45.5,59 45.5,51.78 C19.-
V_ACT  (via drill 0.6)
  Top 0.406: v55.5,5 48.5,5 47.5,4 13.5,4 11.5,6 11.5,27.5 12,28 15.5,28 16,28.5 16,35 16.62,35.62 US4.1 | US2.8 12.88,79.38 10.5,77 10.5,71 6,66.5 6,56 6.5,55.5 11,55.5 11.5,55 v11.5,54 | v11.5,51 11.5,45 12.5,44 R32.1
  Bottom 0.406: J4.6 63,5 62,6 56.5,6 v55.5,5 | v11.5,54 v11.5,51
  Bottom 1.27: US4.1 18.88,35.62 17.5,37 R56.2 17.31,41.5 R57.1 R32.1
V_GATE
  Bottom 1.27: C21.1 56.54,45.24 C20.+ 56.28,49.64 D14.C 55,55 57.5,57.5 57.5,62 58.5,63 R44.1
V_SET  (via drill 0.6)
  Top 0.406: US3.3 52.77,15.23 53.5,14.5 58.5,14.5 v61.5,11.5
  Bottom 0.406: v61.5,11.5 63,10 J4.5
V_TEMP  (via drill 0.6)
  Top 1.27: v44.5,97.5 43,96 41.5,94.5 35,94.5 34.5,94 C12.1
  Bottom 1.27: 20.5,85.5 23,83 33.5,83 34.5,84 C12.1 36.73,86.54 R10.2 | 20.5,85.5 US2.4 | US2.6 15.42,86.08 16,85.5 20.5,85.5 | NTC1.2 48.73,101.73 v44.5,97.5
VCC
  Bottom 1.27: C8.1 61.92,69
  Bottom 1.778: 66,104.5 T9.D | 34,103.5 T8.D
  Bottom 2.54: D7.C D8.C 77,87.54 | 66,99.5 66,104.5 | 34,99 34,103.5
  Bottom 3.81: C11.+ C10.+ 61.92,69 C9.+ 61.92,87.46 62,87.54 | 66,87.54 62.54,87.54 62,87.54 | 66,87.54 77,87.54 | 66,99.5 66,95 66,87.54 | 62,87.54 61.96,87.54 57,92.5 49,92.5 48,93.5 37.5,93.5 34,97 34,99

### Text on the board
tPlace: - | + | AC | AC | Futrzaczek | + -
